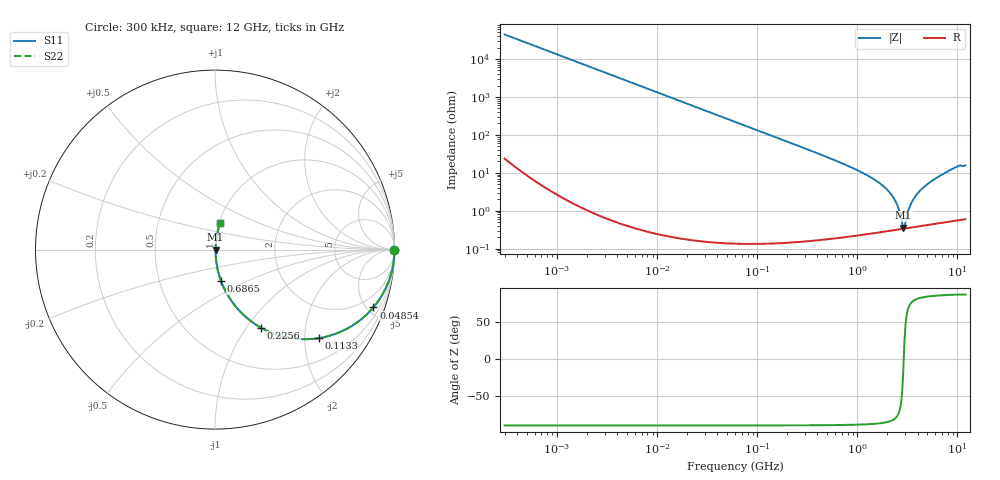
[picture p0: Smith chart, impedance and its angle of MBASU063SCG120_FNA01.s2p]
! MBASU063SCG120_FNA01  S-PARAMETER MODEL  ( General Type )
! Model Generated by TAIYO YUDEN Corporation (http://www.ty-top.com)
! Version 1.0
! TAIYO YUDEN Control No. 130801
! Copyright(c) 2013 TAIYO YUDEN CO.,LTD. All Rights Reserved.
! Product Description (link to TY-COMPAS)
! https://ds.yuden.co.jp/TYCOMPAS/or/detail?pn=MBASU063SCG120JFNA01&u=M
! Products Name : Multilayer Ceramic Capacitors
! Characteristics :
!  Capacitance : 12 pF , Rated Voltage : 50V , TCC : CG / C0G
!  Case Size : 0.6 x 0.3 / 0.024 x 0.012 [mm/inch] , Thickness : 0.3 / 0.012 [mm/inch]
!  (Conditions: Temperature = 25 degC , DC Bias Current/Voltage = 0A / 0V)
! External Node Assignments :
!  1  o---| |---o  2
! GND o---------o GND
! Frequency Range : 0.3MHz  -  12000MHz  [ 401 STEP ]
# MHz S RI R 50
! Freq[MHz].  S11 Real  S11 Imag  S21 Real  S21 Imag  S12 Real  S12 Imag  S22 Real  S22 Imag
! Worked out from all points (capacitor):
!   401 points, 300 kHz to 12 GHz, reference 50 ohm
!   read as one part in series: C = 12 pF near 316.3 kHz
!   lowest |Z| = 354 mohm at 2.87 GHz (marker M1)
!   series resonance near 2.907 GHz, so ESL is about 250 pH
!   S11 on the Smith chart (normalised r, x): 300 kHz: open; 48.54 MHz: 1.00, -5.47; 113.3 MHz: 1.00, -2.34; 225.6 MHz: 1.00, -1.17; 686.5 MHz: 1.00, -0.37; 12 GHz: 1.01, +0.31
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0.3  1 -0.00226  6.3e-06 0.00226  6.3e-06 0.00226  1 -0.00226
1.769972  0.9998 -0.0133  0.000179 0.0133  0.000179 0.0133  0.9998 -0.0133
10.44266  0.9938 -0.0781  0.00615 0.0781  0.00615 0.0781  0.9938 -0.0781
26.39317  0.962 -0.1911  0.038 0.1911  0.038 0.1911  0.962 -0.1911
48.54115  0.8821 -0.3222  0.1179 0.3222  0.1179 0.3222  0.8821 -0.3222
60  0.8304 -0.375  0.1696 0.375  0.1696 0.375  0.8304 -0.375
113.3117  0.5782 -0.4933  0.4218 0.4933  0.4218 0.4933  0.5782 -0.4933
225.6362  0.2557 -0.435  0.7443 0.435  0.7443 0.435  0.2557 -0.435
353.9943  0.1214 -0.3244  0.8786 0.3244  0.8786 0.3244  0.1214 -0.3244
686.4755  0.0341 -0.1762  0.9659 0.1762  0.9659 0.1762  0.0341 -0.1762
1403.667  0.00771 -0.0719  0.9923 0.0719  0.9923 0.0719  0.00771 -0.0719
2088.533  0.00387 -0.0306  0.9961 0.0306  0.9961 0.0306  0.00387 -0.0306
2448.343  0.00337 -0.0157  0.9966 0.0157  0.9966 0.0157  0.00337 -0.0157
2795.104  0.00331 -0.00359  0.9967 0.00359  0.9967 0.00359  0.00331 -0.00359
2870.14  0.00334 -0.00116  0.9967 0.00116  0.9967 0.00116  0.00334 -0.00116
3026.31  0.00342 0.00359  0.9966 -0.00359  0.9966 -0.00359  0.00342 0.00359
3276.641  0.00364 0.0107  0.9964 -0.0107  0.9964 -0.0107  0.00364 0.0107
3547.679  0.00395 0.0176  0.9961 -0.0176  0.9961 -0.0176  0.00395 0.0176
4502.883  0.00556 0.0391  0.9944 -0.0391  0.9944 -0.0391  0.00556 0.0391
8503.825  0.0189 0.1159  0.9811 -0.1159  0.9811 -0.1159  0.0189 0.1159
10236.47  0.0279 0.1474  0.9721 -0.1474  0.9721 -0.1474  0.0279 0.1474
12000  0.0294 0.1509  0.9706 -0.1509  0.9706 -0.1509  0.0294 0.1509
